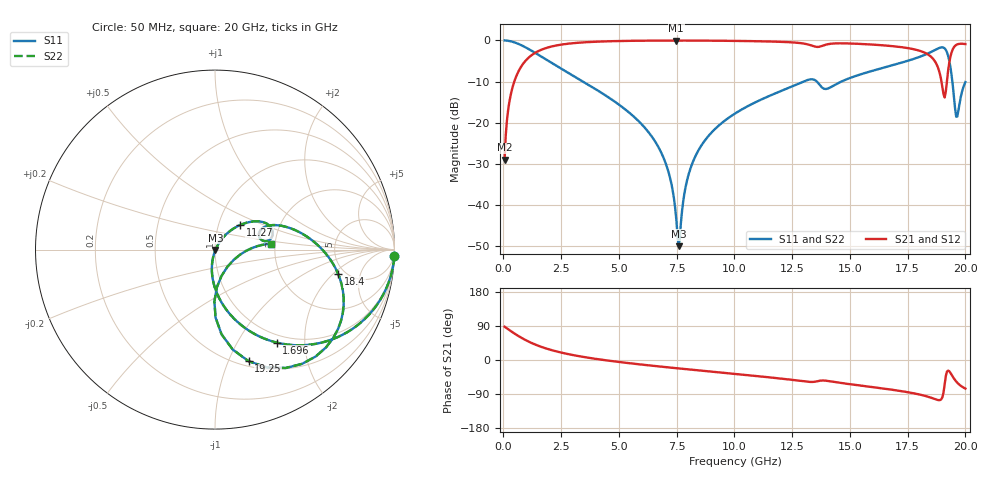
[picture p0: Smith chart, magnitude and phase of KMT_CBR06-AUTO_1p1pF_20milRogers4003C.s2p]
! Data measured by Modelithics Inc. support@modelithics.com 813-866-6335
! KEMET CBR06-AUTO 1.1pF, Pad Width= 0.851mm, Pad Length= 0.64mm, Pad Gap= 0.62mm, 20mil Rogers 4003C substrate Data, January 2022
# hz S ma R 50
! 2 Port Network Data from SP1.SP block
! freq  magS11  angS11  magS21  angS21  magS12  angS12  magS22  angS22
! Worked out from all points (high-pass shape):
!   401 points, 50 MHz to 20 GHz, reference 50 ohm
!   highest |S21| = -0.03 dB at 7.481 GHz (marker M1); lowest = -29.0 dB at 50 MHz (marker M2)
!   |S21| within 3 dB of the highest: 1.369 GHz to 18.26 GHz (16.89 GHz wide, 172 % of centre); 19.4 GHz to end of sweep
!   lowest |S11| = -50.1 dB at 7.581 GHz (marker M3), VSWR 1.01, Z = 50.3 - j0.163 ohm
!   |S11| at or under -10 dB: 3.442 GHz to 12.99 GHz (9.548 GHz wide, 116 % of centre); 13.57 GHz to 14.63 GHz (1.067 GHz wide, 7.57 % of centre); 19.43 GHz to end of sweep
!   |S22| runs from -50.1 to 0.0 dB; largest |S21 - S12| = 0
!   S11 on the Smith chart (normalised r, x): 50 MHz: 1, -53; 1.696 GHz: 0.88, -1.48; 11.27 GHz: 1.27, +0.36; 18.4 GHz: 4.37, -2.32; 19.25 GHz: 0.55, -1.19; 20 GHz: 1.89, +0.14
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5e7  0.9994 -2.2  0.03538 87.8  0.03538 87.8  0.9994 -2.2
2.495e8  0.9846 -10.8  0.1741 79.2  0.1741 79.2  0.9846 -10.8
5.4875e8  0.9313 -22.9  0.3635 67.0  0.3635 67.0  0.9313 -22.9
1.695875e9  0.622 -56.4  0.7814 33.5  0.7814 33.5  0.622 -56.4
3.391625e9  0.3223 -80.8  0.9443 8.8  0.9443 8.8  0.3223 -80.8
6.73325e9  0.04898 -103.6  0.9957 -17.0  0.9957 -17.0  0.04898 -103.6
7.232e9  0.02022 -101.5  0.9965 -20.1  0.9965 -20.1  0.02022 -101.5
7.481375e9  0.00675 -84.5  0.9966 -21.6  0.9966 -21.6  0.00675 -84.5
7.581125e9  0.003141 -31.1  0.9966 -22.2  0.9966 -22.2  0.003141 -31.1
7.93025e9  0.01884 55.9  0.9964 -24.3  0.9964 -24.3  0.01884 55.9
8.32925e9  0.04007 58.6  0.9956 -26.7  0.9956 -26.7  0.04007 58.6
1.0025e10  0.129 51.5  0.9873 -36.7  0.9873 -36.7  0.129 51.5
1.127188e10  0.1973 44.2  0.9745 -44.3  0.9745 -44.3  0.1973 44.2
1.336662e10  0.337 18.0  0.8625 -57.9  0.8625 -57.9  0.337 18.0
1.4015e10  0.2583 18.7  0.8959 -55.0  0.8959 -55.0  0.2583 18.7
1.670825e10  0.4876 10.9  0.8591 -77.5  0.8591 -77.5  0.4876 10.9
1.8404e10  0.6994 -11.2  0.6685 -97.3  0.6685 -97.3  0.6994 -11.2
1.890275e10  0.816 -32.9  0.3846 -105.7  0.3846 -105.7  0.816 -32.9
1.910225e10  0.8006 -52.6  0.2022 -64.5  0.2022 -64.5  0.8006 -52.6
1.925188e10  0.6496 -73.2  0.4294 -27.9  0.4294 -27.9  0.6496 -73.2
1.9601e10  0.1181 -54.2  0.8813 -56.7  0.8813 -56.7  0.1181 -54.2
2e10  0.3118 6.0  0.9044 -75.5  0.9044 -75.5  0.3118 6.0
